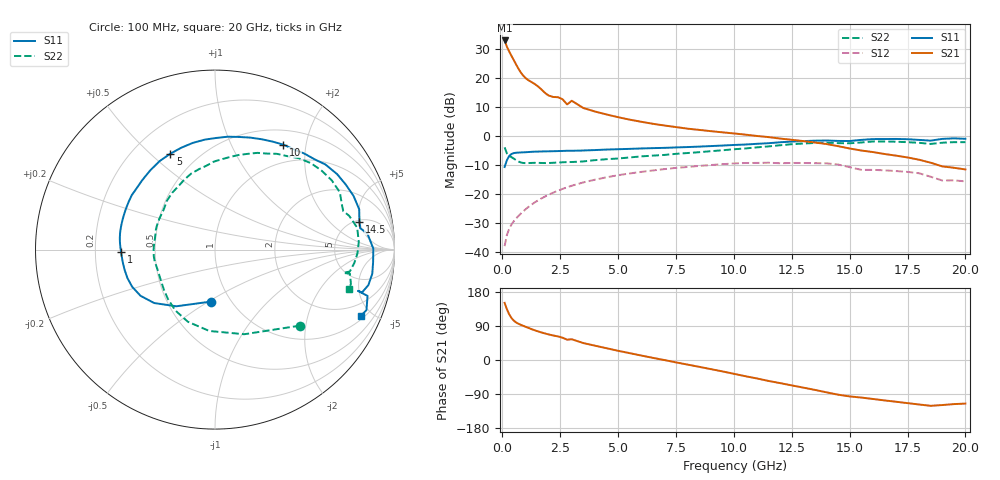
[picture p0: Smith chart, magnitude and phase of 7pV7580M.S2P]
! Infineon Technologies  Discrete & RF Semiconductors
! bfp620
! VCE = 0.75 V,  IC =  80 mA
! Common Emitter S-Parameters:  Sep 2002
# GHz  S  MA  R  50
!  f  S11  S21  S12  S22
! GHz  MAG  ANG  MAG  ANG  MAG  ANG  MAG  ANG
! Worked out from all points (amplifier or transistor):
!   59 points, 100 MHz to 20 GHz, reference 50 ohm
!   highest |S21| = 33.0 dB at 100 MHz (marker M1)
!   |S21| within 3 dB of that: start of sweep to 248.6 MHz
!   unconditionally stable (mu >= 1): 1.651 GHz to 11.48 GHz; 16.36 GHz to end of sweep
!   at 1 GHz: K = 0.96, MSG = 22.7 dB, |S12| = -25.4 dB
!   at 5.5 GHz: K = 1.08, MAG = 7.6 dB, |S12| = -13.0 dB
!   at 20 GHz: K = 1.63, MAG = -2.6 dB, |S12| = -15.7 dB
!   S11 on the Smith chart (normalised r, x): 100 MHz: 0.81, -0.51; 1 GHz: 0.31, -0.01; 5 GHz: 0.35, +0.58; 10 GHz: 0.71, +1.61; 14.5 GHz: 5.24, +5.00; 20 GHz: 1.20, -4.31
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0.1  0.2905 -94.5  44.46 150.7  0.0125 53.1  0.6353 -41.8
0.2  0.3823 -124.3  34.57 133.8  0.0196 52.0  0.499 -70.9
0.3  0.4511 -138.7  28.5 120.3  0.0251 52.3  0.4545 -94.0
0.4  0.4884 -148.2  23.98 110.5  0.0297 53.1  0.4295 -110.6
0.5  0.5058 -155.8  20.2 103.7  0.0338 54.0  0.4047 -123.1
0.6  0.513 -162.0  17.02 99.0  0.0377 54.9  0.3808 -133.4
0.8  0.5183 -171.7  12.46 92.8  0.0456 56.3  0.3484 -149.4
1  0.5234 -178.3  10.02 87.9  0.0539 56.9  0.339 -160.1
1.4  0.5347 172.6  7.882 78.4  0.0711 56.2  0.343 -173.3
2  0.5425 159.9  4.982 67.5  0.0964 52.4  0.3408 168.4
2.6  0.5503 150.5  4.313 58.9  0.1217 47.1  0.3505 157.5
2.8  0.5542 146.7  3.497 53.6  0.1297 45.1  0.3536 151.8
3  0.5537 144.4  4.045 54.8  0.1381 43.1  0.3545 151.1
3.5  0.5604 136.3  3.033 44.7  0.1576 37.7  0.3628 141.9
5  0.5895 115.0  2.106 24.3  0.21 21.5  0.4078 119.9
7  0.6223 89.2  1.513 -0.1  0.2675 0.2  0.4698 95.8
10  0.6978 56.9  1.104 -36.4  0.3349 -33.4  0.5886 66.3
10.5  0.7109 51.7  1.052 -42.8  0.3411 -40.1  0.6081 61.6
13.5  0.8278 21.2  0.77 -78.9  0.3385 -74.6  0.7563 30.7
14.5  0.82 11.0  0.666 -91.5  0.3209 -89.8  0.7504 19.7
17  0.8866 -8.7  0.457 -110.1  0.2476 -105.1  0.7941 -1.5
20  0.8919 -24.4  0.264 -115.0  0.1642 -116.3  0.7802 -16.5
